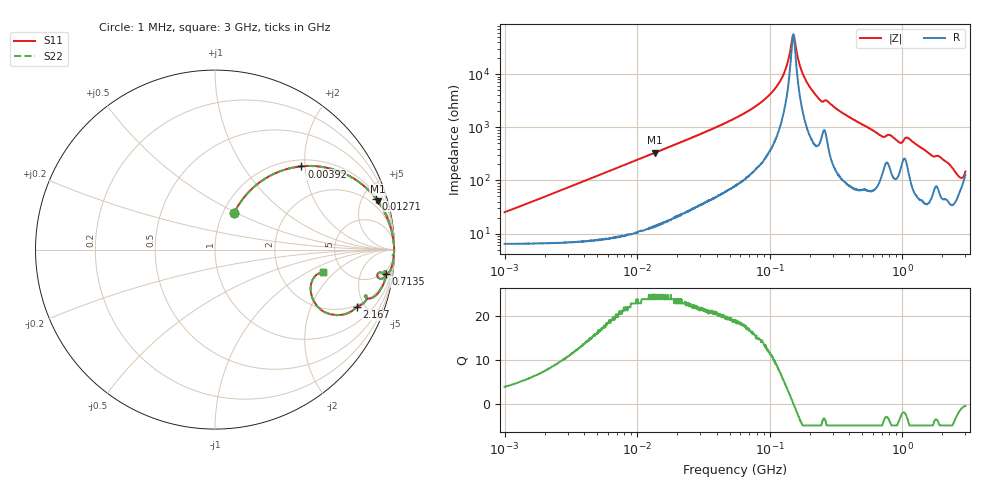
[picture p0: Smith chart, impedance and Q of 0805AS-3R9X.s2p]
!s-Parameter Generated by FASTRON Sdn. Bhd.
!FASTRON P/N : 0805AS-3R9X
!Keysight Technologies: E4991B_MY54100416_A.01.15
!Date: Mon Jun 15 12:59:02 2026
!Version  :Rev01  Mon Jun 15 12:59:02 2026
!Data & Calibration Information:
!Freq  S11  S21  S12  S22
!PortZ  Port1:50+j0  Port2:50+j0
!When reading reference impedance value at option line is always used.
! Remarks : This data is being provided solely for informational purposes.
# Hz S dB R 50
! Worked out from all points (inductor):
!   1601 points, 1 MHz to 3 GHz, reference 50 ohm
!   read as one part in series: L = 3.9 uH near 1.041 MHz
!   highest Q = 24.8 at 13.63 MHz (marker M1), where L = 3.88 uH
!   self-resonance near 150.5 MHz
!   S11 on the Smith chart (normalised r, x): 1 MHz: 1.13, +0.49; 3.92 MHz: 1.14, +1.92; 12.71 MHz: 1.25, +6.21; 713.5 MHz: 4, -13; 2.167 GHz: 1.86, -4.36; 3 GHz: 3.56, -1.45
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1000000  -12.70 62.4  -0.76 -13.0  -0.76 -13.0  -12.70 62.4
1955280  -7.67 58.0  -1.35 -24.2  -1.35 -24.2  -7.67 58.0
3804036  -3.64 44.7  -3.04 -41.0  -3.04 -41.0  -3.64 44.7
3919980  -3.50 43.9  -3.15 -41.8  -3.15 -41.8  -3.50 43.9
1.270533e7  -0.53 17.6  -10.40 -70.0  -10.40 -70.0  -0.53 17.6
1.362733e7  -0.47 16.5  -10.90 -71.2  -10.90 -71.2  -0.47 16.5
1.447069e7  -0.42 15.6  -11.40 -72.1  -11.40 -72.1  -0.42 15.6
5.504702e7  -0.05 3.8  -23.50 -83.2  -23.50 -83.2  -0.05 3.8
8.29729e7  -0.03 2.1  -28.90 -84.1  -28.90 -84.1  -0.03 2.1
1.114693e8  -0.02 1.0  -35.00 -82.8  -35.00 -82.8  -0.02 1.0
1.308271e8  -0.02 0.5  -41.50 -77.2  -41.50 -77.2  -0.02 0.5
1.505037e8  -0.02 0.0  -54.90 -4.6  -54.90 -4.6  -0.02 0.0
1.748812e8  -0.02 -0.5  -41.10 77.5  -41.10 77.5  -0.02 -0.5
2.083556e8  -0.02 -1.1  -34.10 82.3  -34.10 82.3  -0.02 -1.1
2.433181e8  -0.05 -1.8  -30.10 77.8  -30.10 77.8  -0.05 -1.8
7.135306e8  -0.36 -8.1  -16.80 69.8  -16.80 69.8  -0.36 -8.1
7.925923e8  -0.38 -7.3  -17.60 67.3  -17.60 67.3  -0.38 -7.3
9.585869e8  -0.59 -10.0  -14.90 63.9  -14.90 63.9  -0.59 -10.0
1.097256e9  -0.46 -8.2  -16.50 65.9  -16.50 65.9  -0.46 -8.2
2.167021e9  -1.39 -22.1  -8.33 56.7  -8.33 56.7  -1.39 -22.1
2.530652e9  -2.77 -29.4  -5.82 44.3  -5.82 44.3  -2.77 -29.4
3e9  -4.22 -11.9  -7.59 17.7  -7.59 17.7  -4.22 -11.9
